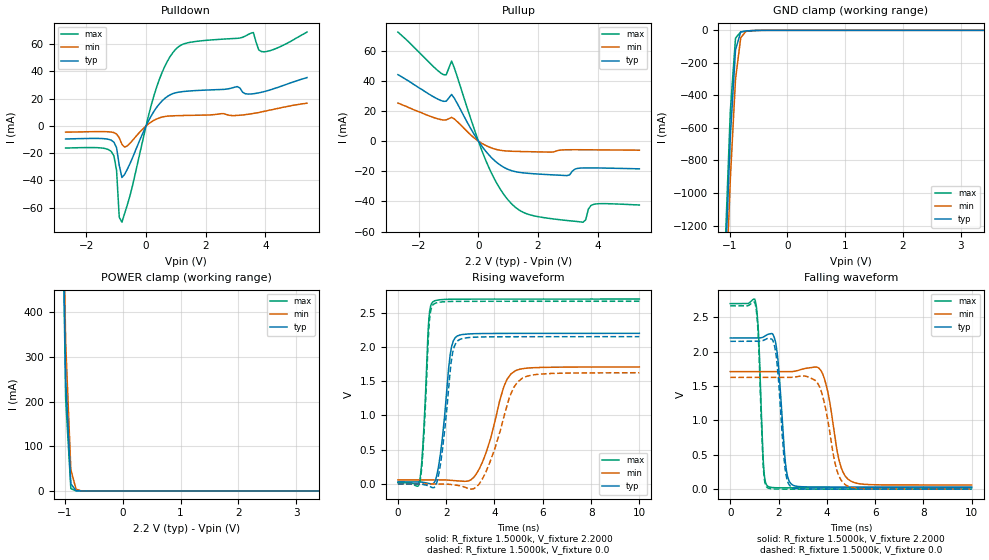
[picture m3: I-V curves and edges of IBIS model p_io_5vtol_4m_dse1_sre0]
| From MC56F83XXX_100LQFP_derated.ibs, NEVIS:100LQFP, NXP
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[Model] p_io_5vtol_4m_dse1_sre0
|   Model p_io_5vtol_4m_dse1_sre0
| Library cells for typ/min/max conditions are connected as defined below:
|  pad - External Pad
|  ipp_do - Core Input
|  ipp_obe - Output Buffer Enable
|  esd_boost - vdd_s_3v
|  esd_bus - vdd_s_3v
|  ipp_ame - vss_s_lv
|  ipp_dse - vdd_s_lv
|  ipp_ina40a_5vtol - NC
|  ipp_ina40b_5vtol - NC
|  ipp_ina_5vtol - NC
|  ipp_ina_mux_3v - NC
|  ipp_ind - NC
|  ipp_ind_3v - NC
|  ipp_pue - vss_s_lv
|  ipp_sre - vss_s_lv
|  tie_3v - vdd_s_3v
|  tie_hi - vdd_s_lv
|  vbuf_3v - vdd_s_3v
|  vdd_bulk_lv - vdd_s_lv
|  vdd_s_3v - vdd_s_3v
|  vdd_s_lv - vdd_s_lv
|  vss_bulk - vss_s_3v
|  vss_s_3v - vss_s_3v
|  vss_s_lv - vss_s_lv
| All other pins connected to ground
Model_type I/O
Polarity   Non-Inverting
Enable   Active-High
Vinl =   0.7700V
Vinh =   1.5400V
Vmeas =  1.1000V
Cref =   25.0000pF
Rref =   1.0000k
Vref =   0.0V
C_comp   2.5897pF   2.5141pF   2.6932pF
[Temperature Range]   25.0000   0.1250k   -40.0000
[Voltage Range]   2.2000V   1.7100V   2.7000V
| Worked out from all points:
|   slope of the pulldown table from 0 to 0.33 V, typ, clamps not added: 25.7 ohm
|   slope of the pullup table from 0 to 0.33 V, typ, clamps not added: 38.3 ohm
|   GND clamp passes 1 mA (typ) near -0.56 V on its own axis
|   POWER clamp passes 1 mA (typ) near -0.81 V on its own axis
|   rising waveform, R_fixture 1.5000k, V_fixture 2.2000: 20-80 % time 357ps typ, 774ps min, 207ps max; typ from 0.031 V to 2.2 V
|   rising waveform, R_fixture 1.5000k, V_fixture 0.0: 20-80 % time 368ps typ, 842ps min, 213ps max; typ from 0 V to 2.15 V
|   falling waveform, R_fixture 1.5000k, V_fixture 2.2000: 20-80 % time 259ps typ, 472ps min, 164ps max; typ from 2.2 V to 0.032 V
|   falling waveform, R_fixture 1.5000k, V_fixture 0.0: 20-80 % time 266ps typ, 512ps min, 164ps max; typ from 2.15 V to 0.001 V
[Pulldown]
|Voltage   I(typ)   I(min)   I(max)
-2.7V     -9.58mA    -4.57mA    -16.24mA
-1.17V    -10.45mA   -4.486mA   -18.73mA
-990mV    -15.98mA   -5.899mA   -32.6mA
-900mV    -28.96mA   -8.728mA   -67.1mA
-810mV    -37.86mA   -13.49mA   -70.68mA
270mV     10.92mA    4.187mA    22.64mA
990mV     24.34mA    7.491mA    56.19mA
3.06V     28.9mA     7.71mA     64.33mA
3.6V      23.63mA    9.2mA      68.56mA
3.78V     24.28mA    9.8mA      55.81mA
4.05V     25.71mA    11.1mA     54.67mA
5.4V      35.5mA     16.7mA     68.9mA
[Pullup]
|Voltage   I(typ)   I(min)   I(max)
-2.7V     44mA       25.2mA     72.2mA
-1.17V    26.34mA    13.97mA    43.99mA
-1.08V    26.42mA    14.03mA    43.92mA
-900mV    30.88mA    15.71mA    53mA
360mV     -9.303mA   -3.93mA    -17.88mA
810mV     -16.87mA   -6.301mA   -34.14mA
1.35V     -20.64mA   -6.862mA   -45.44mA
2.97V     -22.84mA   -5.752mA   -52.58mA
3.51V     -17.79mA   -5.736mA   -53.71mA
3.69V     -17.74mA   -5.75mA    -45.02mA
3.87V     -17.76mA   -5.78mA    -41.87mA
5.4V      -18.37mA   -6.03mA    -42.34mA
[GND_clamp]
|Voltage   I(typ)   I(min)   I(max)
-2.7V     -20.35A    -20.38A    -20.37A
-1.08V    -1.486A    -1.737A    -1.339A
-990mV    -654.8mA   -915.7mA   -496.6mA
-900mV    -120.3mA   -300.6mA   -47.98mA
-810mV    -10.43mA   -45.61mA   -9.206mA
-720mV    -3.577mA   -6.172mA   -6.342mA
-540mV    -682.6uA   -563.7uA   -1.265mA
5.4V      0A         0A         0A
[POWER_clamp]
|Voltage   I(typ)   I(min)   I(max)
-2.7V     20.23A     19.96A     20.45A
-1.08V    950.5mA    990.2mA    948mA
-990mV    252.7mA    333.8mA    206.6mA
-900mV    16.05mA    47.59mA    5.278mA
-810mV    508.3uA    3.841mA    61.17uA
-720mV    15.33uA    281.3uA    694.4nA
-630mV    461.8nA    20.43uA    7.955nA
5.4V      0A         0A         0A
[Ramp]
| variable   typ   min   max
dV/dt_r  0.6013/0.6303n   0.2061/1.0273n   1.0878/0.3490n
dV/dt_f  0.7290/0.3945n   0.2308/0.5522n   1.2634/0.2266n
R_load = 50.0000
[Rising Waveform]
R_fixture= 1.5000k
V_fixture= 2.2000
V_fixture_min= 1.7100
V_fixture_max= 2.7000
|time   V(typ)   V(min)   V(max)
0s        31.17mV    60.02mV    18.84mV
919.5ps   30.78mV    60.01mV    91.53mV
1.282ns   8.226mV    60.09mV    2.413V
1.447ns   3.959mV    60.27mV    2.659V
1.758ns   435.1mV    60.48mV    2.69V
2.169ns   1.9V       54.09mV    2.697V
2.459ns   2.16V      45.47mV    2.698V
3.365ns   2.196V     217.8mV    2.699V
4.869ns   2.199V     1.655V     2.699V
10ns      2.199V     1.708V     2.7V
[Rising Waveform]
R_fixture= 1.5000k
V_fixture= 0.0
V_fixture_min= 0.0
V_fixture_max= 0.0
|time   V(typ)   V(min)   V(max)
0s        554.5pV    116.8nV    15.42pV
925ps     -422.4uV   -11.58uV   53.71mV
1.296ns   -31.52mV   76.09uV    2.353V
1.461ns   -54.01mV   295.3uV    2.619V
1.698ns   153.9mV    642.5uV    2.652V
2.196ns   1.759V     -7.306mV   2.665V
2.486ns   2.094V     -20.73mV   2.666V
3.477ns   2.147V     59.83mV    2.667V
5.162ns   2.15V      1.547V     2.667V
10ns      2.151V     1.624V     2.667V
[Falling Waveform]
R_fixture= 1.5000k
V_fixture= 2.2000
V_fixture_min= 1.7100
V_fixture_max= 2.7000
|time   V(typ)   V(min)   V(max)
0s        2.2V       1.71V      2.7V
1.054ns   2.2V       1.71V      2.712V
1.378ns   2.215V     1.71V      342.1mV
1.534ns   2.249V     1.71V      48.36mV
1.907ns   2.075V     1.71V      21.05mV
2.282ns   395.9mV    1.709V     19.8mV
2.523ns   76.4mV     1.711V     19.62mV
3.755ns   32.34mV    1.726V     19.35mV
4.981ns   31.9mV     120.2mV    19.29mV
10ns      31.69mV    61.08mV    19.18mV
[Falling Waveform]
R_fixture= 1.5000k
V_fixture= 0.0
V_fixture_min= 0.0
V_fixture_max= 0.0
|time   V(typ)   V(min)   V(max)
0s        2.151V     1.626V     2.668V
1.036ns   2.151V     1.626V     2.693V
1.371ns   2.165V     1.626V     306.7mV
1.533ns   2.192V     1.626V     23.56mV
1.871ns   2.021V     1.626V     2.171mV
2.263ns   324.8mV    1.626V     928.9uV
2.513ns   34.93mV    1.627V     748.9uV
3.68ns    1.097mV    1.504V     496.2uV
4.791ns   728.7uV    59.37mV    439.6uV
10ns      501.2uV    942.9uV    324.1uV
